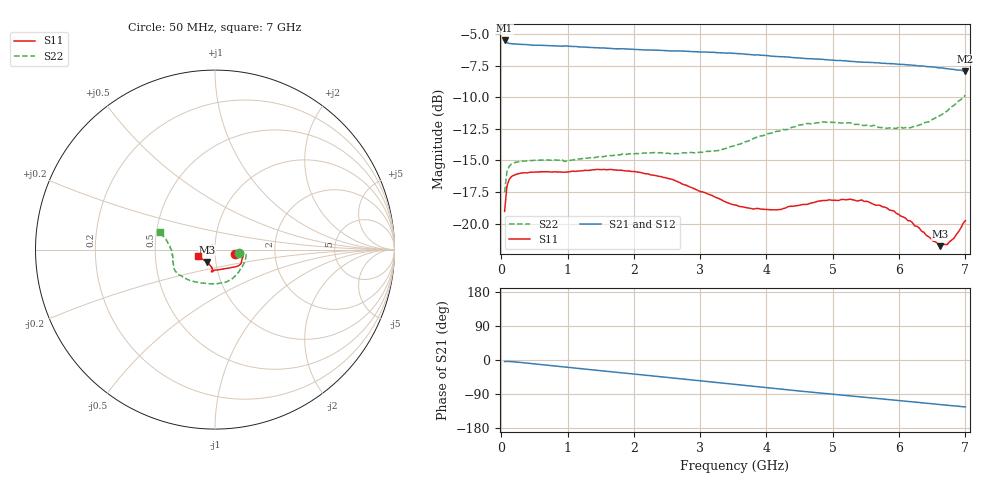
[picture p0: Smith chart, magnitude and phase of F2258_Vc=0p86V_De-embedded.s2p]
! Integrated Device Technology
! Corporate Headquarters
! 6024 Silver Creek Valley Road
! San Jose, CA 95138  USA
! Phone:  1-408-284-8200
! Toll Free:  1-800-223-1366
! Webpage:  http://www.idt.com/
! Timing and RF Division
! 515 Groton Road, Suite 102
! Westford, MA 01886-6024
! Device:  F2258
! Description: Voltage Variable RF Attenuator
! Frequency:  50.0 -  6000.00 MHz
! Package:  3x3 mm Thin QFN Plastic Package: 16 pin
! Ports:  2 RF, 2 DC
!  Pin  1  = NC
!  Pin  2  = NC
!  Pin  3  = RF2  = Port 2
!  Pin  4  = GND
!  Pin  5  = Vdd
!  Pin  6  = NC
!  Pin  7  = VCTRL
!  Pin  8  = NC
!  Pin  9  = GND
!  Pin 10  = RF1  = Port 1
!  Pin 11  = NC
!  Pin 12  = NC
!  Pin 13  = NC
!  Pin 14  = NC
!  Pin 15  = NC
!  Pin 16  = NC
! Vcntrl:  0.860 Volts
! Vdd:  +3.300 Volts
! Current:  1.141 mA
! Data:  The device was measured on a the F2258 evaluation board which has
!  individual transmission lines to the RF pins.  Data was collected
!  using a calibrated network analyzer.  The evaluation board was
!  de-embedded using a TRL calibration technique.
!  The reference plane is the edge of the package pin.
! Misc:  SN 10
!  Action Tracker AT0285
! Date Measured:  2014-12-10
! Date:  2016-01-13  MJV
! Note:
!  Integrated Device Technology supplies this data as a sample of measured
!  data at the package pin for this product.  Your particular data for this
!  product may vary.
!  Data was taken at 25 degrees C.
!  Integrated Device Technology reserves the right to change this data at anytime.
!Freq_(GHz)  S11M_(dB)  S11P_(deg)  S21M_(dB)  S21P_(deg)  S12M_(dB)  S12P_(deg)  S22M_(dB)  S22P_(deg)
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# GHz S dB R 50
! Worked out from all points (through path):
!   201 points, 50 MHz to 7 GHz, reference 50 ohm
!   highest |S21| = -5.52 dB at 50 MHz (marker M1); lowest = -8.0 dB at 7 GHz (marker M2)
!   group delay of S21, straight-line fit = 48.8 ps
!   lowest |S11| = -21.8 dB at 6.618 GHz (marker M3), VSWR 1.18, Z = 45.4 - j6.27 ohm
!   |S11| at or under -10 dB: start of sweep to end of sweep
!   |S22| runs from -17.5 to -9.8 dB; largest |S21 - S12| = 0.0025
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0.05  -19.02 -11.2  -5.52 -4.2  -5.50 -4.2  -17.51 -9.2
0.08475  -17.05 -6.1  -5.68 -3.7  -5.68 -3.7  -15.88 -6.2
0.1195  -16.49 -4.9  -5.75 -3.9  -5.73 -3.9  -15.45 -6.3
0.15425  -16.26 -4.8  -5.77 -4.3  -5.76 -4.3  -15.27 -7.2
0.5365  -15.91 -11.2  -5.90 -10.8  -5.87 -10.8  -14.97 -19.0
0.9535  -15.92 -20.2  -5.95 -18.5  -5.95 -18.5  -15.08 -33.5
1.2315  -15.81 -24.2  -6.03 -23.5  -6.02 -23.5  -14.84 -42.3
1.6485  -15.70 -29.4  -6.14 -30.9  -6.13 -30.9  -14.61 -54.1
2.37825  -16.25 -36.9  -6.29 -43.7  -6.33 -43.7  -14.39 -73.9
2.93425  -17.29 -46.2  -6.41 -53.7  -6.43 -53.7  -14.41 -92.2
3.525  -18.51 -64.9  -6.53 -64.5  -6.54 -64.5  -13.82 -115.5
3.803  -18.84 -76.2  -6.66 -69.5  -6.64 -69.5  -13.26 -126.0
4.1505  -18.90 -87.8  -6.78 -75.7  -6.76 -75.7  -12.69 -136.5
4.7065  -18.33 -98.2  -6.98 -85.4  -6.96 -85.4  -12.08 -149.4
5.2625  -18.06 -99.1  -7.17 -94.7  -7.16 -94.7  -12.02 -158.5
5.43625  -18.12 -97.5  -7.22 -97.6  -7.23 -97.6  -12.21 -161.4
5.85325  -18.91 -96.4  -7.35 -104.5  -7.35 -104.6  -12.43 -169.9
6.166  -19.76 -99.5  -7.45 -109.8  -7.47 -109.8  -12.42 -177.1
6.61775  -21.77 -122.7  -7.68 -117.5  -7.69 -117.5  -11.45 170.9
6.722  -21.66 -132.3  -7.74 -119.3  -7.74 -119.3  -11.11 168.1
6.82625  -21.15 -142.6  -7.80 -121.0  -7.80 -121.0  -10.65 166.1
7  -19.75 -158.8  -7.95 -123.7  -7.95 -123.8  -9.84 162.5
